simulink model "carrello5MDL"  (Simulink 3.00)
settings: Solver=ode45  SolverMode=SingleTasking  StartTime=0.0  StopTime=10.0  RelTol=1e-6  AbsTol=1e-7
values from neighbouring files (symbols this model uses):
  b1 = 2*1500*N/(m/sec)    (= 3000)    [carrello2.M]    (also in carrello3.M; carrello4.M; carrello5.M; carrello6.M)
  b2 = 2*1500*N/(m/sec)    (= 3000)    [carrello2.M]    (also in carrello3.M; carrello4.M; carrello5.M; carrello6.M)
  K = 0.8*1800*N/cm    (= 144000)    [carrello2.M]    (also in carrello3.M; carrello4.M; carrello5.M; carrello6.M)
  Ka = KK(1)    [carrello5.M]    (also in carrello6.M)
  Kb = KK(2)    [carrello5.M]    (also in carrello6.M)
  Kc = KK(3)    [carrello5.M]    (also in carrello6.M)
  Kd = KK(4)    [carrello5.M]    (also in carrello6.M)
  Kp = 2*1800*N/cm    (= 360000)    [carrello2.M]    (also in carrello3.M; carrello4.M; carrello5.M; carrello6.M)
  Kr = 1    [carrello5.M]    (also in carrello6.M)
  Ma = 3850*Kg    (= 3850)    [carrello2.M]    (also in carrello3.M; carrello4.M; carrello5.M; carrello6.M)
  mr = 2*134*Kg+524*Kg    (= 792)    [carrello2.M]    (also in carrello3.M; carrello4.M; carrello5.M; carrello6.M)
  R = 1    [carrello4.M]    (also in carrello5.M = 0.1; carrello6.M = 0.1)
  X_12_0 = -Mag/K    (= -0.26228125)    [carrello2.M]    (also in carrello3.M = 0; carrello4.M = 0; carrello5.M = 0; carrello6.M = 0)
  X_20_0 = -(Mag+mrg)/Kp    (= -0.1264945)    [carrello2.M]    (also in carrello3.M = 0; carrello4.M = 0; carrello5.M = 0; carrello6.M = 0)
  Xsdot = 0    [carrello3.M]    (also in carrello4.M; carrello5.M; carrello6.M)

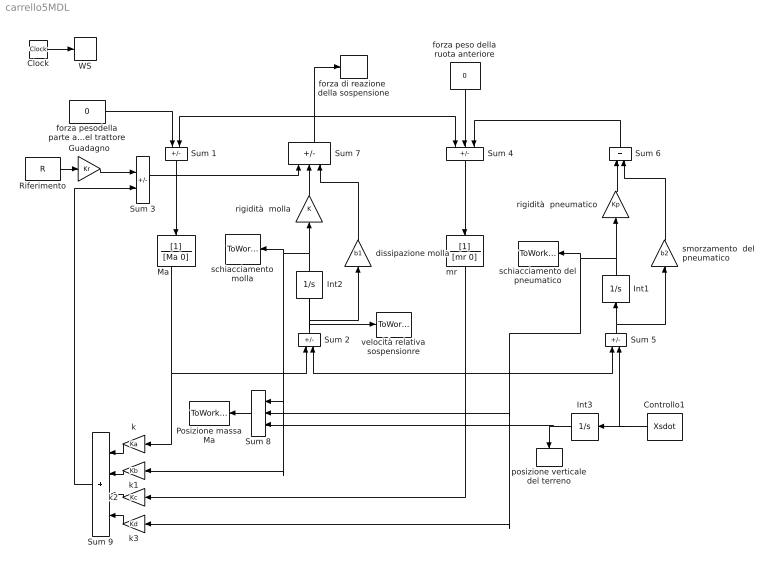
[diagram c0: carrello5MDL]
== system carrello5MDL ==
  Clock : Clock
  Controllo1 : Constant  Orientation=left  Value=Xsdot
  Guadagno : Gain  Gain=Kr  SaturateOnIntegerOverflow=on
  Int1 : Integrator  Orientation=up  ExternalReset=none  InitialConditionSource=internal  InitialCondition=X_20_0  LimitOutput=off  UpperSaturationLimit=inf  LowerSaturationLimit=-inf  ShowSaturationPort=off  ShowStatePort=off  AbsoluteTolerance=auto
  Int2 : Integrator  Orientation=up  ExternalReset=none  InitialConditionSource=internal  InitialCondition=X_12_0  LimitOutput=off  UpperSaturationLimit=inf  LowerSaturationLimit=-inf  ShowSaturationPort=off  ShowStatePort=off  AbsoluteTolerance=auto
  Int3 : Integrator  Orientation=left  ExternalReset=none  InitialConditionSource=internal  InitialCondition=X_20_0  LimitOutput=off  UpperSaturationLimit=inf  LowerSaturationLimit=-inf  ShowSaturationPort=off  ShowStatePort=off  AbsoluteTolerance=auto
  Ma : TransferFcn  Orientation=down  Numerator=[1]  Denominator=[Ma 0]
  Posizione massa Ma : ToWorkspace  VariableName=X_Ma  SampleTime=-1  SaveFormat=Matrix
  Riferimento : Constant  Value=R
  Sum 1 : Sum  Orientation=down  Inputs=+-  SaturateOnIntegerOverflow=on
  Sum 2 : Sum  Orientation=up  Inputs=+-
  Sum 3 : Sum  Inputs=+-
  Sum 4 : Sum  Orientation=down  Inputs=++-
  Sum 5 : Sum  Orientation=up  Inputs=+-
  Sum 6 : Sum  Orientation=up  Inputs=++
  Sum 7 : Sum  Orientation=up  Inputs=-++
  Sum 8 : Sum  Orientation=left  Inputs=+++
  Sum 9 : Sum  Orientation=left  Inputs=++++
  WS : ToWorkspace  VariableName=t  SampleTime=-1  SaveFormat=Matrix
  dissipazione molla : Gain  Orientation=up  Gain=b1  SaturateOnIntegerOverflow=on
  forza di reazione  della sospensione : ToWorkspace  VariableName=R  SampleTime=-1  SaveFormat=Matrix
  forza peso della ruota anteriore : Constant  Orientation=down  Value=0
  forza pesodella parte anteriore del trattore : Constant  Value=0
  k : Gain  Orientation=left  Gain=Ka  SaturateOnIntegerOverflow=on
  k1 : Gain  Orientation=left  Gain=Kb  SaturateOnIntegerOverflow=on
  k2 : Gain  Orientation=left  Gain=Kc  SaturateOnIntegerOverflow=on
  k3 : Gain  Orientation=left  Gain=Kd  SaturateOnIntegerOverflow=on
  mr : TransferFcn  Orientation=down  Numerator=[1]  Denominator=[mr 0]
  posizione verticale del terreno : ToWorkspace  VariableName=Xs  SampleTime=-1  SaveFormat=Matrix
  rigidità  molla : Gain  Orientation=up  Gain=K  SaturateOnIntegerOverflow=on
  rigidità  pneumatico : Gain  Orientation=up  Gain=Kp  SaturateOnIntegerOverflow=on
  schiacciamento del pneumatico : ToWorkspace  VariableName=X_20  SampleTime=-1  SaveFormat=Matrix
  schiacciamento molla : ToWorkspace  VariableName=X_12  SampleTime=-1  SaveFormat=Matrix
  smorzamento  del pneumatico : Gain  Orientation=up  Gain=b2  SaturateOnIntegerOverflow=on
  velocità relativa sospensionre : ToWorkspace  VariableName=vel_rel  SampleTime=-1  SaveFormat=Matrix
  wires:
  forza pesodella parte anteriore del trattore/1 -> Sum 1/1
  Sum 1/1 -> Ma/1
  forza peso della ruota anteriore/1 -> Sum 4/2
  Sum 4/1 -> mr/1
  mr/1 -> Sum 5/1, Sum 2/2, k2/1
  Int1/1 -> rigidità  pneumatico/1, schiacciamento del pneumatico/1, Sum 8/2, k3/1
  Sum 5/1 -> Int1/1, smorzamento  del pneumatico/1
  rigidità  pneumatico/1 -> Sum 6/1
  smorzamento  del pneumatico/1 -> Sum 6/2
  Sum 7/1 -> Sum 1/2, forza di reazione  della sospensione/1, Sum 4/1
  Sum 6/1 -> Sum 4/3
  Sum 2/1 -> velocità relativa sospensionre/1, Int2/1, dissipazione molla/1
  Int2/1 -> rigidità  molla/1, schiacciamento molla/1, Sum 8/1, k1/1
  dissipazione molla/1 -> Sum 7/3
  rigidità  molla/1 -> Sum 7/2
  Controllo1/1 -> Int3/1, Sum 5/2
  Int3/1 -> Sum 8/3, posizione verticale del terreno/1
  Clock/1 -> WS/1
  Sum 8/1 -> Posizione massa Ma/1
  Ma/1 -> Sum 2/1, k/1
  k/1 -> Sum 9/1
  k1/1 -> Sum 9/2
  k2/1 -> Sum 9/3
  k3/1 -> Sum 9/4
  Sum 9/1 -> Sum 3/2
  Sum 3/1 -> Sum 7/1
  Riferimento/1 -> Guadagno/1
  Guadagno/1 -> Sum 3/1
